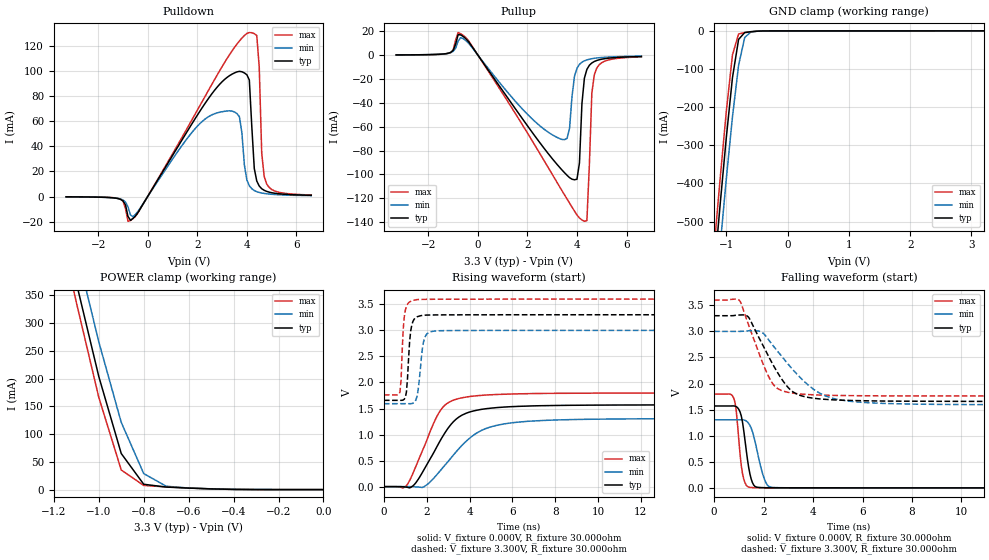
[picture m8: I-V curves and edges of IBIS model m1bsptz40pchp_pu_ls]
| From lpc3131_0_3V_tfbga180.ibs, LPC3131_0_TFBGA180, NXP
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| |   Rev 0.20 IBIS Model Design Automation Generation   |
| |   N O N - S I L I C O N   C O R R E L A T E D   |
| |   This IBIS [Model] is pre-Beta tactical support   |
| |  Note: this IBIS [Model] contains clamp curves generated   |
| |   through simulation which should not be relied upon   |
| Date/Time   : 2010 Jan 25 (Mon) 11:58:19
| Pccmos090 jliolib_p50 2.0
|   0.9 um 3.3V pad library
|   seven level metal
|   dual oxide
|   dual threshold voltage
|   nominal line mixed supply
|   parasitic extracted netlists
| Process block a10
| mem1bsptz40pchp
|   Bidirectional Pad 3.3
|   3state Output
|   Plain Input
|   CMOS
|   Programmable between
|   - (p1=0, p2=1) plain input
|   - (p1=0, p2=0) with Pull Up
|   - (p1=1, p2=1) with Pull Down
|   - (p1=1, p2=0) with Repeater
| Pull Up Mode low speed (esh=1, p1=0, p2=0)
[Model]   m1bsptz40pchp_pu_ls | of mem1bsptz40pchp
Model_type   I/O
Polarity   Non-Inverting
Enable   Active-Low
|  Reciever Thresholds
Vinl   = 0.99V
Vinh   = 2.31V
| AC Test Load Conditions
Vref   = 0
Cref   = 0
Rref   = 1000000000
Vmeas   = 1.65
| [Process Range]   typical   min   max
| C_comp edge width   400.000ps   400.000ps   400.000ps
| C_comp Tstrobe   40.000fs   40.000fs   40.000fs
C_comp   200.000pF   200.000pF   200.000pF
[Temperature Range]   25   125   -40
[Voltage Range]   3.30V   3.00V   3.60V
[GND Clamp Reference]   0.00V   0.00V   0.00V
[Pulldown Reference]   0.00V   0.00V   0.00V
[POWER Clamp Reference]   3.30V   3.00V   3.60V
[Pullup Reference]   3.30V   3.00V   3.60V
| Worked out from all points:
|   slope of the pulldown table from 0 to 0.495 V, typ, clamps not added: 30.7 ohm
|   slope of the pullup table from 0 to 0.495 V, typ, clamps not added: 33.4 ohm
|   GND clamp passes 1 mA (typ) near -0.51 V on its own axis
|   POWER clamp passes 1 mA (typ) near -0.47 V on its own axis
|   rising waveform, V_fixture 0.000V, R_fixture 30.000ohm: 20-80 % time 1.41ns typ, 1.86ns min, 1.14ns max; typ from 0.001 V to 1.57 V
|   falling waveform, V_fixture 0.000V, R_fixture 30.000ohm: 20-80 % time 280ps typ, 398ps min, 217ps max; typ from 1.57 V to 0.001 V
|   rising waveform, V_fixture 3.300V, R_fixture 30.000ohm: 20-80 % time 163ps typ, 221ps min, 137ps max; typ from 1.66 V to 3.3 V
|   falling waveform, V_fixture 3.300V, R_fixture 30.000ohm: 20-80 % time 1.17ns typ, 1.67ns min, 897ps max; typ from 3.3 V to 1.66 V
[GND Clamp]
| ref voltage   0.00V   0.00V   0.00V
|   Voltage   I(typ)   I(min)   I(max)
-3.3V     -4.732A    -4.814A    -4.684A
-1.2V     -636mA     -742.5mA   -569.7mA
-1.1V     -453.5mA   -561.8mA   -385.7mA
-1V       -279mA     -387.5mA   -210.8mA
-900mV    -122.8mA   -225.5mA   -63.15mA
-800mV    -22.47mA   -90.5mA    -8.27mA
-700mV    -4.437mA   -17.32mA   -4.624mA
-600mV    -2.227mA   -3.085mA   -2.65mA
-300mV    -253.1uA   -168.6uA   -385.4uA
3.2V      -17.82uA   34.39uA    -87.56uA
[Power Clamp]   | Vtable = Vcc - Vpad
| ref voltage   3.30V   3.00V   3.60V
|   Voltage   I(typ)   I(min)   I(max)
-3.3V     4.647A     4.675A     4.636A
-1.2V     553.3mA    610.4mA    520.8mA
-1.1V     373.2mA    433.6mA    337.9mA
-1V       204mA      266.6mA    166.4mA
-900mV    65.07mA    121.2mA    35.4mA
-800mV    9.632mA    28.93mA    7.456mA
-700mV    4.576mA    6.079mA    4.901mA
-600mV    2.711mA    2.826mA    2.897mA
-400mV    366.5uA    549.1uA    304.5uA
0V        388.1pA    9.875nA    264.4pA
[Pulldown]
| ref voltage   0.00V   0.00V   0.00V
|   Voltage   I(typ)   I(min)   I(max)
-3.3V     -237uA     -253uA     -192.2uA
-1.2V     -1.654mA   -1.559mA   -1.497mA
-600mV    -17.52mA   -16.02mA   -17.7mA
2.8V      87.36mA    66.79mA    96.99mA
3.7V      99.96mA    63.73mA    124.2mA
4.1V      93mA       8.514mA    130.9mA
4.3V      22.4mA     4.741mA    130.1mA
4.4V      12.38mA    3.859mA    128.6mA
4.5V      8.362mA    3.243mA    103.4mA
4.6V      6.217mA    2.791mA    34.69mA
4.8V      4.107mA    2.175mA    10.04mA
6.6V      975.1uA    710uA      1.215mA
[Pullup]   | Vtable = Vcc - Vpad
| ref voltage   3.30V   3.00V   3.60V
|   Voltage   I(typ)   I(min)   I(max)
-3.3V     206.8uA    209.1uA    174.1uA
-500mV    14.05mA    12.42mA    15mA
3.4V      -96.4mA    -70.68mA   -113.8mA
3.7V      -102.7mA   -61.3mA    -124.1mA
3.9V      -104.5mA   -17.66mA   -130.8mA
4.1V      -90.31mA   -7.691mA   -136.5mA
4.2V      -40.65mA   -5.885mA   -138.2mA
4.3V      -19.22mA   -4.74mA    -139.3mA
4.4V      -11.93mA   -3.955mA   -138.7mA
4.6V      -6.527mA   -2.958mA   -31.83mA
4.7V      -5.3mA     -2.623mA   -16.4mA
6.6V      -1.122mA   -812.7uA   -1.418mA
[Ramp]
R_load   = 30.000ohm
|   dV/dt(typ)   dV/dt(min)   dV/dt(max)
dV/dt_r   941.410mV/1.400ns   782.844mV/1.850ns   1.078V/1.100ns
dV/dt_f   985.619mV/1.150ns   844.091mV/1.700ns   1.103V/900.000ps
[Rising Waveform]  | cubic spline decimation from 501 points
V_fixture   = 0.000V
R_fixture   = 30.000ohm
|   Time   V(typ)   V(min)   V(max)
0s        906.1uV    713.4uV    1.177mV
900ps     -2.483mV   737.2uV    -22.48mV
1.35ns    14.3mV     -1.14mV    252.1mV
1.9ns     347.5mV    6.232mV    788.6mV
2.65ns    898.3mV    316.1mV    1.469V
3.25ns    1.249V     609.3mV    1.661V
3.85ns    1.411V     875.1mV    1.721V
5ns       1.507V     1.149V     1.764V
7.3ns     1.554V     1.268V     1.789V
25ns      1.57V      1.305V     1.798V
[Falling Waveform]  | cubic spline decimation from 501 points
V_fixture   = 0.000V
R_fixture   = 30.000ohm
|   Time   V(typ)   V(min)   V(max)
0s        1.57V      1.305V     1.798V
800ps     1.571V     1.305V     1.715V
900ps     1.557V     1.305V     1.459V
1.05ns    1.456V     1.306V     646.7mV
1.15ns    1.258V     1.306V     268.5mV
1.45ns    265.2mV    1.196V     10.51mV
1.65ns    29.88mV    899.7mV    4.339mV
2ns       4.318mV    214.4mV    2.438mV
2.35ns    2.293mV    10.47mV    2.011mV
25ns      906.2uV    713.5uV    1.177mV
[Rising Waveform]  | cubic spline decimation from 501 points
V_fixture   = 3.300V
V_fixture_min = 3.000V
V_fixture_max = 3.600V
R_fixture   = 30.000ohm
|   Time   V(typ)   V(min)   V(max)
0s        1.657V     1.593V     1.761V
750ps     1.657V     1.593V     1.821V
800ps     1.657V     1.593V     2.049V
900ps     1.664V     1.593V     3.023V
1ns       1.715V     1.593V     3.387V
1.25ns    2.988V     1.593V     3.558V
1.5ns     3.25V      1.671V     3.588V
1.85ns    3.29V      2.781V     3.596V
2.35ns    3.296V     2.987V     3.598V
25ns      3.3V       3V         3.6V
[Falling Waveform]  | cubic spline decimation from 501 points
V_fixture   = 3.300V
V_fixture_min = 3.000V
V_fixture_max = 3.600V
R_fixture   = 30.000ohm
|   Time   V(typ)   V(min)   V(max)
0s        3.3V       3V         3.6V
1ns       3.313V     3V         3.604V
1.35ns    3.291V     3.01V      3.183V
1.95ns    2.754V     2.976V     2.412V
2.35ns    2.389V     2.747V     2.011V
2.6ns     2.184V     2.599V     1.895V
3.15ns    1.854V     2.285V     1.818V
4.4ns     1.7V       1.784V     1.778V
6ns       1.671V     1.639V     1.766V
25ns      1.657V     1.593V     1.761V
